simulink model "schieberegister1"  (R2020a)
settings: Solver=VariableStepDiscrete  StartTime=0.0  StopTime=Inf  RelTol=1e-3  EnableMultiTasking=on

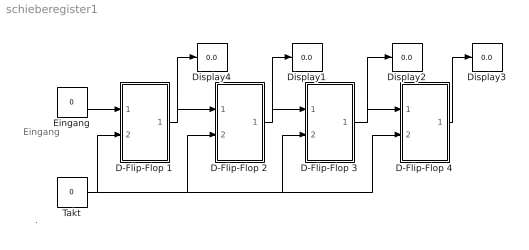
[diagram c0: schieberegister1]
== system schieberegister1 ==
  note: Eingang
  note: .
  D-Flip-Flop 1 : Subsystem  mask(DFlipFlop){s0=off}
      mask prompts: s0 "Initially on"
      mask help: D Flip-Flop Block
  D-Flip-Flop 2 : Subsystem  mask(DFlipFlop){s0=off}
      mask prompts: s0 "Initially on"
      mask help: D Flip-Flop Block
  D-Flip-Flop 3 : Subsystem  mask(DFlipFlop){s0=off}
      mask prompts: s0 "Initially on"
      mask help: D Flip-Flop Block
  D-Flip-Flop 4 : Subsystem  mask(DFlipFlop){s0=off}
      mask prompts: s0 "Initially on"
      mask help: D Flip-Flop Block
  Display{1..4} (4 alike) : Display
  Eingang : Constant  Value=0  OutDataTypeStr=double
  Takt : Constant  Value=0  OutDataTypeStr=double
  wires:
  D-Flip-Flop 1/1(Q) -> D-Flip-Flop 2/1(D), Display4/1
  D-Flip-Flop 2/1(Q) -> D-Flip-Flop 3/1(D), Display1/1
  D-Flip-Flop 3/1(Q) -> D-Flip-Flop 4/1(D), Display2/1
  Eingang/1 -> D-Flip-Flop 1/1(D)
  Takt/1 -> D-Flip-Flop 1/2(CLK), D-Flip-Flop 2/2(CLK), D-Flip-Flop 3/2(CLK), D-Flip-Flop 4/2(CLK)
  D-Flip-Flop 4/1(Q) -> Display3/1

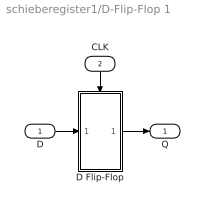
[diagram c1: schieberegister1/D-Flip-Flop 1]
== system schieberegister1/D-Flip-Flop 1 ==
  D : Inport
  CLK : Inport  Port=2
  D Flip-Flop : Subsystem  TreatAsAtomicUnit=on
  Q : Outport  InitialOutput=0
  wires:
  CLK/1 -> D Flip-Flop/Trigger
  D Flip-Flop/1(Q) -> Q/1
  D/1 -> D Flip-Flop/1(D)

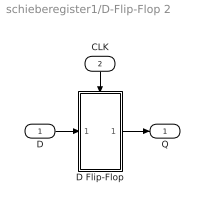
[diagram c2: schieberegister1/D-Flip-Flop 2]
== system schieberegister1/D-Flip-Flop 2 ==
  D : Inport
  CLK : Inport  Port=2
  D Flip-Flop : Subsystem  TreatAsAtomicUnit=on
  Q : Outport  InitialOutput=0
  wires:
  D/1 -> D Flip-Flop/1(D)
  D Flip-Flop/1(Q) -> Q/1
  CLK/1 -> D Flip-Flop/Trigger

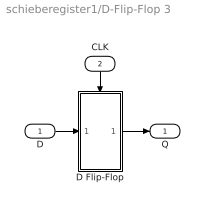
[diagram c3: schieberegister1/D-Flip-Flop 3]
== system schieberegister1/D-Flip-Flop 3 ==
  D : Inport
  CLK : Inport  Port=2
  D Flip-Flop : Subsystem  TreatAsAtomicUnit=on
  Q : Outport  InitialOutput=0
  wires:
  CLK/1 -> D Flip-Flop/Trigger
  D Flip-Flop/1(Q) -> Q/1
  D/1 -> D Flip-Flop/1(D)

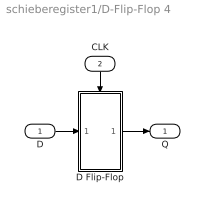
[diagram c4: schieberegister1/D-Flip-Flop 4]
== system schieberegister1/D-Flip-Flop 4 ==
  D : Inport
  CLK : Inport  Port=2
  D Flip-Flop : Subsystem  TreatAsAtomicUnit=on
  Q : Outport  InitialOutput=0
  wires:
  D/1 -> D Flip-Flop/1(D)
  D Flip-Flop/1(Q) -> Q/1
  CLK/1 -> D Flip-Flop/Trigger

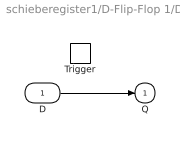
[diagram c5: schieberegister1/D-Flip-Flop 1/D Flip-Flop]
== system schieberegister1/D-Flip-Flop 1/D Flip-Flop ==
  D : Inport
  Trigger : TriggerPort  TriggerType=falling  VariantControl=Variant
  Q : Outport  InitialOutput=s0
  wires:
  D/1 -> Q/1

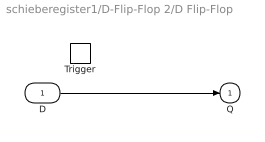
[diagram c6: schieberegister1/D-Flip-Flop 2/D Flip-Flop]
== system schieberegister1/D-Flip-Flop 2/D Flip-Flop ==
  D : Inport
  Trigger : TriggerPort  TriggerType=falling  VariantControl=Variant
  Q : Outport  InitialOutput=s0
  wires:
  D/1 -> Q/1

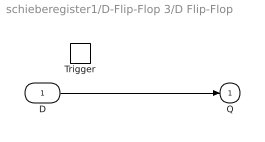
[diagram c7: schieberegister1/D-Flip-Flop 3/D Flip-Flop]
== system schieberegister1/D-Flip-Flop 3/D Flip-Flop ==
  D : Inport
  Trigger : TriggerPort  TriggerType=falling  VariantControl=Variant
  Q : Outport  InitialOutput=s0
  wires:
  D/1 -> Q/1

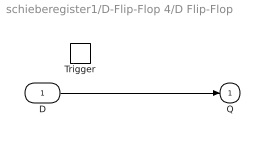
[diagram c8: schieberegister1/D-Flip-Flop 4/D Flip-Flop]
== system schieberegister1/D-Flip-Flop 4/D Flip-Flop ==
  D : Inport
  Trigger : TriggerPort  TriggerType=falling  VariantControl=Variant
  Q : Outport  InitialOutput=s0
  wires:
  D/1 -> Q/1
